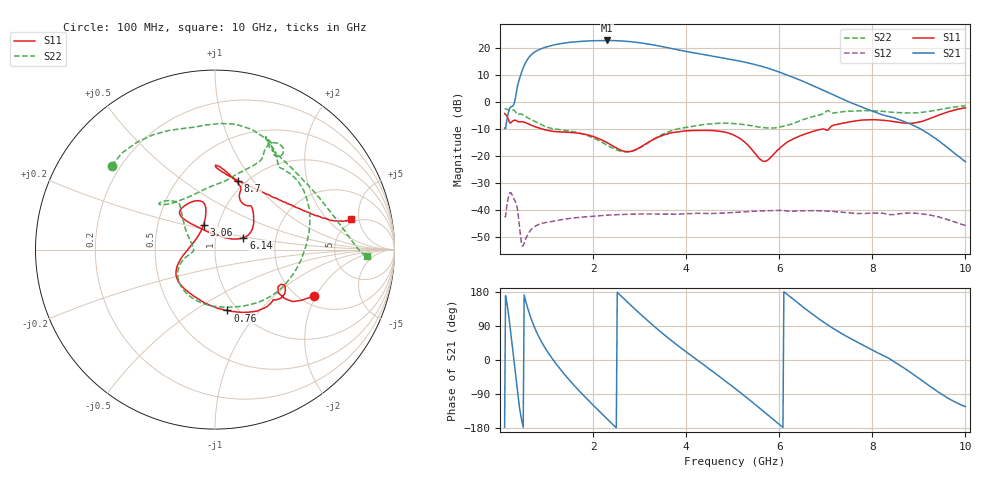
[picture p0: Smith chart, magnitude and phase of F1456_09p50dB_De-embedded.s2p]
! Integrated Device Technology
! Corporate Headquarters
! 6024 Silver Creek Valley Road
! San Jose, CA 95138  USA
! Phone:  1-408-284-8200
! Toll Free:  1-800-223-1366
! Webpage:  http://www.idt.com/
! Timing and RF Division
! 515 Groton Road, Suite 102
! Westford, MA 01886-6024
! Device:  F1456
! Description: 6-bit 0.5 dB Transmit Variable Gain Amplifier
! Frequency:  2100.0 -  2950.00 MHz
! Package:  6x6 mm Thin QFN Plastic Package: 28 pin
! State:  19
! Atten State:  9.5 dB
! Voltage:  +5.00 Volts
! Current:  217.014 mA
! Data:  The device was measured on a the F1455 evaluation board which has
!  individual transmission lines to the RF pins.  Data was collected
!  using a calibrated network analyzer.  The evaluation board was
!  de-embedded using a TRL calibration technique.
!  The reference plane is the edge of the package pin.
!  Pin  1 = CSb
!  Pin  2 = DATA
!  Pin  3 = CLK
!  Pin  4 = RSET
!  Pin  5 = GND
!  Pin  6 = RFIN  = Port 1
!  Pin  7 = GND
!  Pin  8 = NC
!  Pin  9 = NC
!  Pin 10 = NC
!  Pin 11 = NC
!  Pin 12 = NC
!  Pin 13 = NC
!  Pin 14 = /STBY
!  Pin 15 = GND
!  Pin 16 = RFOUT  = Port 2
!  Pin 17 = GND
!  Pin 18 = NC
!  Pin 19 = NC
!  Pin 20 = NC
!  Pin 21 = GND
!  Pin 22 = NC
!  Pin 23 = GND
!  Pin 24 = NC
!  Pin 25 = NC
!  Pin 26 = NC
!  Pin 27 = GND
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# GHz S dB R 50
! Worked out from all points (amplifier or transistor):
!   496 points, 100 MHz to 10 GHz, reference 50 ohm
!   highest |S21| = 22.7 dB at 2.3 GHz (marker M1)
!   |S21| within 3 dB of that: 895.1 MHz to 3.694 GHz (2.799 GHz wide, 122 % of centre)
!   unconditionally stable (mu >= 1): start of sweep to end of sweep
!   at 1.74 GHz: K = 4.58, MAG = 22.9 dB, |S12| = -42.6 dB
!   at 5.06 GHz: K = 7.54, MAG = 16.3 dB, |S12| = -40.8 dB
!   at 10 GHz: K = 139.91, MAG = -12.7 dB, |S12| = -45.7 dB
!   S11 on the Smith chart (normalised r, x): 100 MHz: 2.34, -1.93; 760 MHz: 0.90, -0.69; 3.06 GHz: 0.85, +0.24; 6.14 GHz: 1.36, +0.19; 8.7 GHz: 0.92, +0.84; 10 GHz: 4.57, +3.88
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0.1  -4.31 -25.2  -9.69 -177.3  -42.31 45.8  -2.59 140.9
0.32  -6.75 -32.6  0.39 -19.7  -36.52 -138.3  -3.36 65.0
0.44  -7.31 -43.7  9.67 -141.1  -49.34 142.2  -4.44 39.3
0.58  -7.92 -59.9  15.40 143.6  -49.62 176.4  -5.72 5.8
0.76  -9.22 -78.5  18.59 81.0  -45.95 133.9  -7.29 -28.1
0.98  -10.34 -100.0  20.20 29.9  -44.61 93.2  -9.15 -64.6
1.2  -11.00 -117.6  21.20 -9.0  -43.94 67.7  -10.07 -93.5
1.5  -11.26 -135.7  22.00 -54.2  -43.10 41.8  -10.78 -124.6
1.76  -11.75 -147.2  22.37 -88.8  -42.60 23.8  -11.76 -143.3
2.02  -12.89 -157.1  22.61 -121.3  -42.22 8.1  -13.43 -156.7
2.3  -15.03 -170.8  22.70 -155.2  -41.89 -7.6  -15.96 -166.9
2.64  -18.13 159.0  22.49 164.4  -41.62 -25.4  -18.40 -176.9
3.06  -16.28 114.4  21.70 116.3  -41.43 -46.5  -16.48 158.7
3.4  -13.05 103.2  20.71 79.7  -41.46 -62.6  -12.86 139.4
4.12  -10.61 114.4  18.26 10.8  -41.31 -92.6  -9.09 129.9
5.06  -12.57 135.4  15.38 -75.8  -40.83 -132.3  -8.04 140.7
5.62  -21.60 88.4  13.15 -131.2  -40.29 -161.0  -9.44 126.2
6.14  -15.29 22.9  10.08 176.1  -40.25 168.0  -8.77 88.5
6.7  -11.07 39.4  6.19 122.2  -40.20 137.2  -5.55 64.6
8.36  -7.03 86.8  -5.41 4.0  -41.65 64.7  -3.77 62.3
8.7  -7.86 71.7  -7.40 -22.8  -41.13 53.9  -4.07 51.2
10  -2.20 12.5  -22.11 -122.8  -45.71 -25.2  -1.46 -2.5
